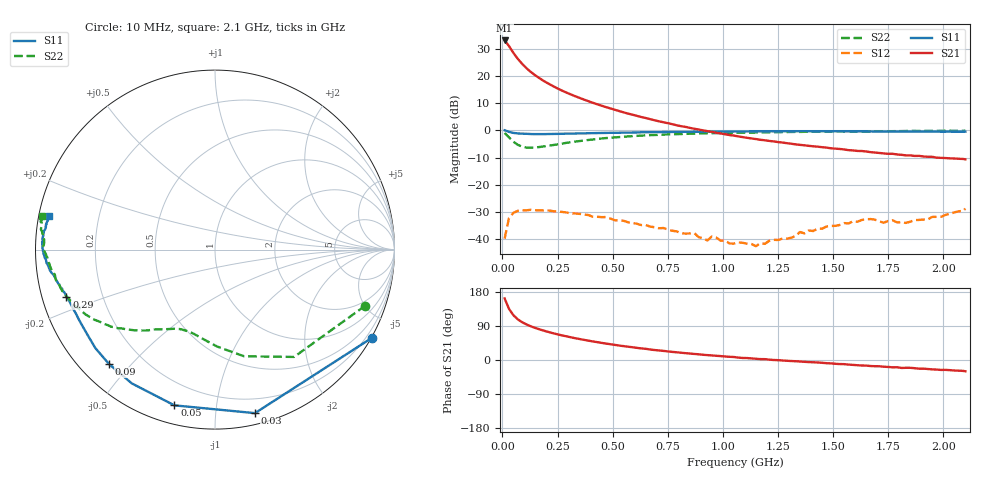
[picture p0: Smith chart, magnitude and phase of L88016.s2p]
!  1/8/97
# MHZ  S  MA  R  50.0000
!  POLYFET RF DEVICES
!  L88016
!  S PARAMETERS
!  VDS=28V, IDQ=200mA
! FREQ  S11MAG  S11ANG  S21MAG  S21ANG  S12MAG  S12ANG  S22MAG  S22ANG
! Date: Wed Jan 08 11:32:39 1997
! SCATTERING PARAMETERS :
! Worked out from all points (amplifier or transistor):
!   106 points, 10 MHz to 2.1 GHz, reference 50 ohm
!   highest |S21| = 33.1 dB at 10 MHz (marker M1)
!   |S21| within 3 dB of that: start of sweep to 37.36 MHz
!   unconditionally stable (mu >= 1): nowhere
!   at 350 MHz: K = 0.15, MSG = 21.3 dB, |S12| = -30.7 dB
!   at 1.07 GHz: K = 0.31, MSG = 19.5 dB, |S12| = -41.2 dB
!   at 2.1 GHz: K = -0.75, MSG = 9.1 dB, |S12| = -28.8 dB
!   S11 on the Smith chart (normalised r, x): 10 MHz: -0.02, -3.82; 30 MHz: 0.08, -1.27; 50 MHz: 0.09, -0.77; 90 MHz: 0.08, -0.43; 290 MHz: 0.07, -0.15; 2.1 GHz: 0.03, +0.10
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10  1.003 -29.4  45.03 162.5  0.01017 64.7  0.8942 -20.4
30  0.9379 -76.3  35.46 134.8  0.02452 44.5  0.7428 -53.6
50  0.8968 -104.6  26.57 118.0  0.03036 29.9  0.6159 -74.8
70  0.8778 -121.9  20.64 107.2  0.03311 19.1  0.5407 -88.7
90  0.8689 -132.8  16.62 99.5  0.03372 12.8  0.5007 -98.1
110  0.8634 -140.5  13.8 93.7  0.03391 7.5  0.4823 -104.8
130  0.8548 -145.8  11.76 88.6  0.0345 2.6  0.4797 -110.0
150  0.8524 -149.9  10.2 84.5  0.03392 -1.5  0.484 -113.8
170  0.8528 -153.0  8.999 80.6  0.03373 -4.1  0.4949 -117.0
190  0.8529 -155.3  7.992 77.1  0.03356 -6.6  0.5079 -119.4
230  0.8582 -158.8  6.496 70.6  0.03257 -11.9  0.5364 -124.2
250  0.8603 -160.3  5.895 67.7  0.03199 -14.4  0.5518 -126.4
290  0.8684 -162.5  4.956 62.5  0.03087 -17.9  0.5886 -130.1
370  0.8787 -165.6  3.675 53.2  0.02833 -25.5  0.65 -136.6
450  0.8943 -167.9  2.841 45.2  0.02532 -30.4  0.7084 -142.4
530  0.9033 -170.1  2.262 38.1  0.02202 -34.9  0.7523 -147.4
710  0.9278 -173.5  1.466 25.2  0.0158 -35.5  0.826 -156.6
1070  0.9565 -178.8  0.7734 6.3  0.00869 -3.5  0.904 -169.9
1150  0.9579 -179.9  0.6914 3.2  0.0074 4.7  0.9133 -172.2
1410  0.9615 176.8  0.5082 -6.0  0.01405 35.1  0.942 -178.4
1770  0.9502 172.3  0.3698 -19.4  0.02215 19.9  0.9654 174.9
2100  0.9441 168.5  0.2928 -29.7  0.03634 13.9  0.9833 169.2
